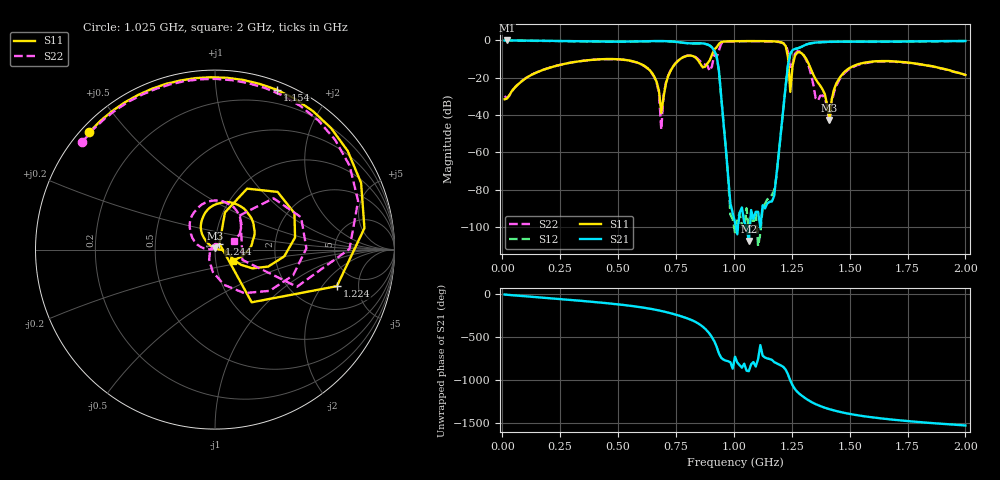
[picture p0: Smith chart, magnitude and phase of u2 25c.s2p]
!Agilent Technologies,E8363B,SG43030131,A.07.50.48
!Agilent E8363B: A.07.50.48
!Date: Tuesday, December 02, 2025 02:25:35
!Correction: S11(Full 2 Port(1,2))
!S21(Full 2 Port(1,2))
!S12(Full 2 Port(1,2))
!S22(Full 2 Port(1,2))
!S2P File: Measurements: S11, S21, S12, S22:
# Hz S  dB  R 50
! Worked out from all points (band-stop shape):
!   201 points, 10 MHz to 2 GHz, reference 50 ohm
!   highest |S21| = 0.01 dB at 19.95 MHz (marker M1); lowest = -107.6 dB at 1.065 GHz (marker M2)
!   |S21| within 3 dB of the highest: start of sweep to 899 MHz; 1.298 GHz to end of sweep
!   lowest |S11| = -42.6 dB at 1.413 GHz (marker M3), VSWR 1.01, Z = 50 + j0.74 ohm
!   |S11| at or under -10 dB: start of sweep to 442.6 MHz; 485 MHz to 768.3 MHz (283.3 MHz wide, 45.2 % of centre); 1.313 GHz to end of sweep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
!   |S22| runs from -47.9 to -0.4 dB; largest |S21 - S12| = 0.017
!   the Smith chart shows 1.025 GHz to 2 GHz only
!   S11 on the Smith chart (normalised r, x): 1.025 GHz: 0.02, +0.39; 1.154 GHz: 0.07, +1.46; 1.224 GHz: 3.44, -2.82; 1.244 GHz: 1.05, +0.07; 2 GHz: 1.22, -0.15
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1e7  -31.57 -80.8  -0.01 -0.8  -0.09 -1.6  -29.80 -79.5
1.995e7  -31.20 -83.8  0.01 -3.5  -0.09 -4.2  -31.03 -87.0
3.483e8  -10.92 -165.9  -0.48 -76.1  -0.56 -76.1  -10.92 -163.2
6.7665e8  -27.02 89.7  -0.30 173.4  -0.38 173.4  -28.19 85.2
6.866e8  -38.78 116.6  -0.31 167.6  -0.39 167.6  -47.91 58.6
7.264e8  -16.36 -137.3  -0.48 141.5  -0.56 141.5  -16.19 -123.4
8.5575e8  -12.63 57.9  -1.53 4.0  -1.60 4.0  -11.33 141.3
9.1545e8  -4.79 -115.9  -5.62 173.6  -5.70 173.6  -7.60 -102.1
9.7515e8  -0.47 169.1  -72.73 -59.7  -73.71 -60.9  -0.62 176.1
1.005e9  -0.40 148.4  -97.67 -6.5  -103.04 -99.4  -0.47 153.1
1.0249e9  -0.37 137.0  -92.42 -105.8  -92.53 -69.4  -0.43 141.1
1.0647e9  -0.34 116.4  -107.63 -175.9  -102.29 -146.3  -0.40 120.2
1.15425e9  -0.40 68.8  -86.60 -33.7  -84.52 -11.9  -0.52 72.7
1.1841e9  -0.57 46.4  -72.13 -82.6  -73.02 -82.3  -0.71 51.4
1.2239e9  -2.99 -16.7  -24.21 -158.0  -24.27 -158.2  -2.51 0.3
1.2438e9  -27.61 53.0  -7.20 75.8  -7.26 75.8  -15.72 -20.7
1.29355e9  -6.92 8.6  -3.25 -102.8  -3.33 -102.8  -6.78 -18.3
1.3433e9  -18.37 -28.3  -1.25 171.9  -1.33 171.8  -23.81 -120.5
1.41295e9  -42.59 92.8  -0.72 99.7  -0.78 99.6  -44.67 132.7
1.47265e9  -17.53 125.9  -0.63 59.2  -0.70 59.1  -18.12 158.0
1.67165e9  -11.07 54.2  -0.66 -18.6  -0.72 -18.7  -11.27 82.3
2e9  -18.52 -30.9  -0.27 -90.4  -0.33 -90.5  -18.53 24.7
